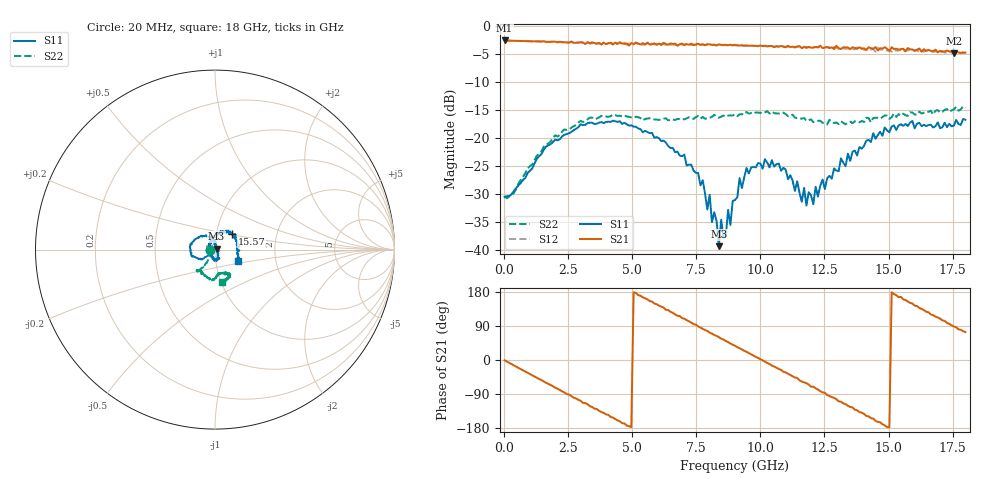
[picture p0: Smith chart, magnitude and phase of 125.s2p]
!Agilent Technologies,N5230A,US43500223,A.07.50.48
!Agilent N5230A: A.07.50.48
!Date: Sunday, January 31, 2016 17:08:56
!Correction: S11(Full 2 Port(1,2))
!S21(Full 2 Port(1,2))
!S12(Full 2 Port(1,2))
!S22(Full 2 Port(1,2))
!S2P File: Measurements: S11, S21, S12, S22:
# Hz S  dB  R 50
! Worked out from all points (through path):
!   201 points, 20 MHz to 18 GHz, reference 50 ohm
!   highest |S21| = -2.66 dB at 20 MHz (marker M1); lowest = -4.9 dB at 17.55 GHz (marker M2)
!   group delay of S21, straight-line fit = 99.6 ps
!   lowest |S11| = -39.3 dB at 8.381 GHz (marker M3), VSWR 1.02, Z = 50.9 + j0.59 ohm
!   |S11| at or under -10 dB: start of sweep to end of sweep
!   |S22| runs from -30.8 to -14.4 dB; largest |S21 - S12| = 0.073
!   S11 on the Smith chart (normalised r, x): 20 MHz: 0.94, -0.00; 15.57 GHz: 1.19, +0.21; 18 GHz: 1.28, -0.17
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2e7  -30.56 -179.7  -2.66 -0.8  -2.66 -1.0  -30.35 179.9
1.5483e9  -22.13 -141.7  -2.79 -56.6  -2.82 -57.0  -21.59 -121.6
3.0766e9  -17.75 -164.1  -3.01 -113.1  -3.06 -112.8  -17.20 -127.1
4.515e9  -17.05 168.0  -3.02 -161.7  -2.93 -164.2  -16.08 -130.6
6.0433e9  -20.08 130.6  -3.21 143.5  -3.44 141.6  -16.82 -125.9
7.7514e9  -27.58 82.9  -3.33 82.1  -3.40 81.0  -16.29 -116.0
7.9312e9  -32.80 76.8  -3.31 76.7  -3.46 74.4  -16.52 -116.4
8.2908e9  -34.82 62.3  -3.56 63.6  -3.49 61.7  -16.31 -113.8
8.3807e9  -39.32 32.4  -3.35 60.3  -3.48 58.1  -16.43 -112.5
8.4706e9  -34.61 4.6  -3.44 56.3  -3.49 55.0  -16.24 -111.8
8.6504e9  -37.63 -24.9  -3.46 50.1  -3.49 48.6  -16.22 -111.2
8.7403e9  -32.85 -20.5  -3.51 47.2  -3.50 45.1  -16.04 -108.8
8.8302e9  -35.53 -38.9  -3.41 43.4  -3.52 41.9  -16.00 -109.0
9.01e9  -31.10 -48.5  -3.43 37.5  -3.55 35.6  -15.83 -106.0
9.4595e9  -25.39 -64.6  -3.56 21.5  -3.58 19.4  -15.40 -100.8
1.01787e10  -23.81 -82.4  -3.60 -4.2  -3.68 -6.8  -15.46 -93.8
1.20666e10  -31.84 170.3  -3.95 -70.2  -3.83 -74.6  -17.22 -83.8
1.35949e10  -22.49 89.8  -3.87 -125.2  -4.22 -131.5  -17.39 -72.2
1.50333e10  -19.02 58.1  -4.55 -177.3  -4.39 176.5  -16.63 -61.3
1.55727e10  -17.88 42.4  -4.14 160.2  -4.70 159.2  -15.71 -58.6
1.75505e10  -17.85 -12.1  -4.92 88.5  -4.73 85.2  -14.94 -70.1
1.8e10  -16.79 -26.6  -4.81 73.8  -4.93 67.8  -14.64 -77.6
